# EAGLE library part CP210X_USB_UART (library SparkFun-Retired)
Single-Chip USB to UART Bridge Source: www.silabs.com .. CP2101.pdf / cp2102.pdf. Spark Fun Electronics SKU : COM-00310 RETIRED: IC-00865
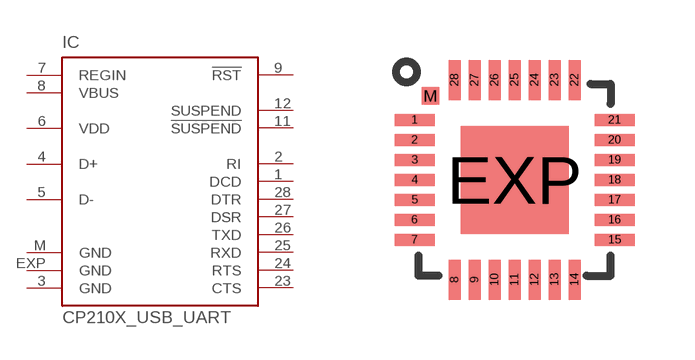
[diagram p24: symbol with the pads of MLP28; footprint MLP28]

Designator prefix IC

## CP210X_USB_UART (PROD_ID: COM-00310; VALUE: CP2101)  [MLP28]
1  DCD  in
2  RI  in
3  GND  pwr
4  D+
5  D-
6  VDD  pwr
7  REGIN  pas
8  VBUS  in
9  !RST
11  !SUSPEND  out
12  SUSPEND  out
23  CTS  in
24  RTS  out
25  RXD  in
26  TXD  out
27  DSR  in
28  DTR  out
EXP  GND  pwr
M  GND  pwr

## Footprint MLP28 (pad centres in mm)
MLP 28 Source: www.silabs.com .. CP2101.pdf
smd 1 x 0.3: 1 -2.5,1.5; 2 -2.5,1; 3 -2.5,0.5; 4 -2.5,0; 5 -2.5,-0.5; 6 -2.5,-1; 7 -2.5,-1.5; 15 2.5,-1.5; 16 2.5,-1; 17 2.5,-0.5; 18 2.5,0; 19 2.5,0.5; 20 2.5,1; 21 2.5,1.5
smd 0.3 x 1: 8 -1.5,-2.5; 9 -1,-2.5; 10 -0.5,-2.5; 11 0,-2.5; 12 0.5,-2.5; 13 1,-2.5; 14 1.5,-2.5; 22 1.5,2.5; 23 1,2.5; 24 0.5,2.5; 25 0,2.5; 26 -0.5,2.5; 27 -1,2.5; 28 -1.5,2.5
smd 2.7 x 2.7: EXP 0,0
smd 0.435 x 0.435: M -2.103,2.103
